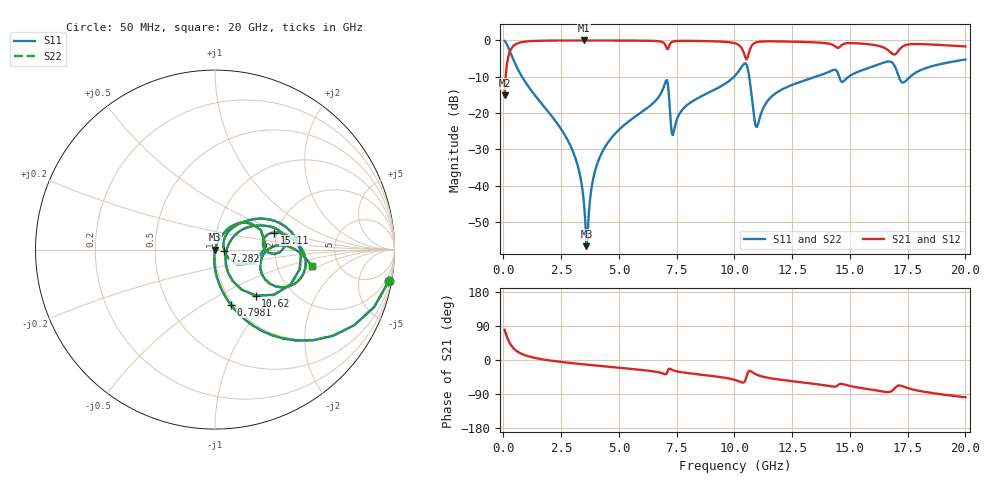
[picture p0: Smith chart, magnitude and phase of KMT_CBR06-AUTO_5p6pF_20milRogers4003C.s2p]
! Data measured by Modelithics Inc. support@modelithics.com 813-866-6335
! KEMET CBR06-AUTO 5.6pF, Pad Width= 0.851mm, Pad Length= 0.64mm, Pad Gap= 0.62mm, 20mil Rogers 4003C substrate Data, January 2022
# hz S ma R 50
! 2 Port Network Data from SP1.SP block
! freq  magS11  angS11  magS21  angS21  magS12  angS12  magS22  angS22
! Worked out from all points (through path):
!   401 points, 50 MHz to 20 GHz, reference 50 ohm
!   highest |S21| = -0.01 dB at 3.491 GHz (marker M1); lowest = -15.2 dB at 50 MHz (marker M2)
!   group delay of S21, straight-line fit = 15.3 ps
!   lowest |S11| = -56.6 dB at 3.591 GHz (marker M3), VSWR 1.00, Z = 50.1 - j0.0997 ohm
!   |S11| at or under -10 dB: 805.2 MHz to 9.981 GHz (9.176 GHz wide, 170 % of centre); 10.64 GHz to 13.53 GHz (2.891 GHz wide, 23.9 % of centre); 17.12 GHz to 17.61 GHz (491.4 MHz wide, 2.83 % of centre)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
!   |S22| runs from -56.6 to -0.1 dB; largest |S21 - S12| = 0
!   S11 on the Smith chart (normalised r, x): 50 MHz: 1, -11; 798.1 MHz: 0.97, -0.66; 7.282 GHz: 1.11, -0.02; 10.62 GHz: 1.33, -0.77; 15.11 GHz: 1.92, +0.41; 20 GHz: 3.16, -0.83
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5e7  0.9846 -10.2  0.1747 79.8  0.1747 79.8  0.9846 -10.2
2.99375e8  0.6828 -47.9  0.73 42.0  0.73 42.0  0.6828 -47.9
7.98125e8  0.3189 -74.0  0.9471 15.9  0.9471 15.9  0.3189 -74.0
2.74325e9  0.04468 -95.4  0.9978 -6.8  0.9978 -6.8  0.04468 -95.4
3.391625e9  0.01021 -94.0  0.9986 -11.0  0.9986 -11.0  0.01021 -94.0
3.491375e9  0.005529 -88.5  0.9986 -11.6  0.9986 -11.6  0.005529 -88.5
3.591125e9  0.001474 -42.4  0.9986 -12.2  0.9986 -12.2  0.001474 -42.4
3.94025e9  0.01488 70.6  0.9984 -14.3  0.9984 -14.3  0.01488 70.6
4.33925e9  0.03173 70.8  0.9979 -16.6  0.9979 -16.6  0.03173 70.8
6.73325e9  0.1688 53.3  0.9731 -32.5  0.9731 -32.5  0.1688 53.3
7.0325e9  0.2778 22.9  0.8342 -37.8  0.8342 -37.8  0.2778 22.9
7.281875e9  0.0538 -10.7  0.9476 -25.4  0.9476 -25.4  0.0538 -10.7
1.0025e10  0.3269 31.6  0.9129 -52.7  0.9129 -52.7  0.3269 31.6
1.0424e10  0.48 -2.3  0.6496 -58.5  0.6496 -58.5  0.48 -2.3
1.06235e10  0.3425 -48.5  0.6699 -29.2  0.6699 -29.2  0.3425 -48.5
1.097262e10  0.06439 -4.3  0.946 -38.9  0.946 -38.9  0.06439 -4.3
1.167088e10  0.1756 36.6  0.9712 -49.2  0.9712 -49.2  0.1756 36.6
1.336662e10  0.3039 26.1  0.9433 -62.2  0.9433 -62.2  0.3039 26.1
1.511225e10  0.3413 16.2  0.917 -70.0  0.917 -70.0  0.3413 16.2
1.670825e10  0.513 -12.9  0.7089 -84.2  0.7089 -84.2  0.513 -12.9
1.730675e10  0.2629 -12.4  0.8329 -69.8  0.8329 -69.8  0.2629 -12.4
2e10  0.5458 -9.7  0.825 -98.4  0.825 -98.4  0.5458 -9.7
